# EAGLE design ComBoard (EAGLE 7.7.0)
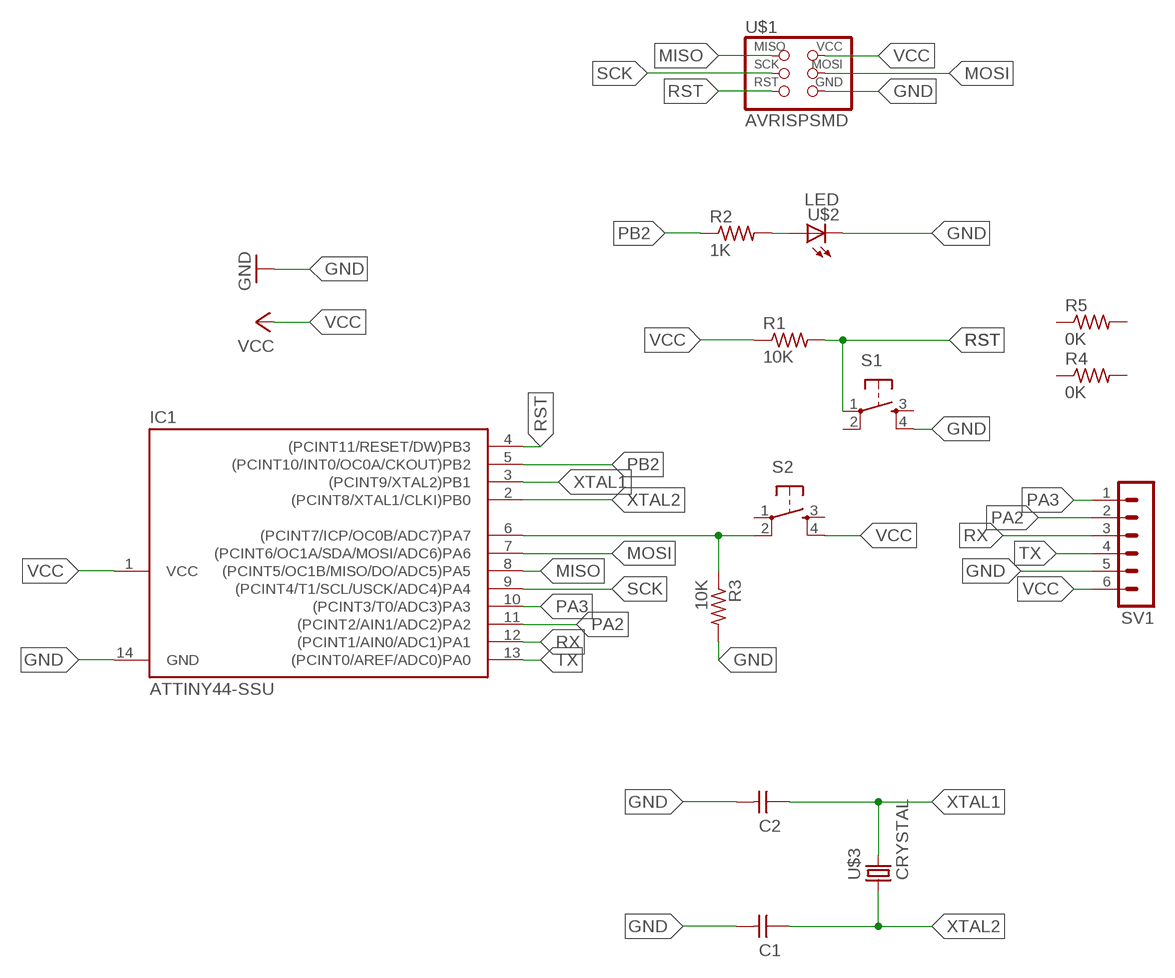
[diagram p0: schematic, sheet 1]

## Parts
C1  CAP-UNPOLARIZED  [C1206]
C2  CAP-UNPOLARIZED  [C1206]
IC1  ATTINY44-SSU  [SOIC14]
R1  10K  RES-US1206  [R1206]
R2  1K  RES-US1206  [R1206]
R3  10K  RES-US1206  [R1206]
R4  0K  RES-US1206  [R1206]
R5  0K  RES-US1206  [R1206]
S1  6MM_SWITCH6MM_SWITCH  [6MM_SWITCH]
S2  6MM_SWITCH6MM_SWITCH  [6MM_SWITCH]
SV1  MA06-1  [MA06-1]
U$1  AVRISPSMD  [2X03SMD]
U$2  LED  [LED1206]
U$3  CRYSTAL  [2-SMD-5X3MM]

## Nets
GND: C1.2 C2.2 IC1.14(GND) R3.2 S1.4(S1) SV1.5 U$1.6(GND) U$2.2(C)
MISO: IC1.8((PCINT5/OC1B/MISO/DO/ADC5)PA5) U$1.1(MISO)
MOSI: IC1.7((PCINT6/OC1A/SDA/MOSI/ADC6)PA6) U$1.4(MOSI)
N$1: R2.2 U$2.1(A)
N$2: IC1.6((PCINT7/ICP/OC0B/ADC7)PA7) R3.1 S2.2(P1)
PA2: IC1.11((PCINT2/AIN1/ADC2)PA2) SV1.2
PA3: IC1.10((PCINT3/T0/ADC3)PA3) SV1.1
PB2: IC1.5((PCINT10/INT0/OC0A/CKOUT)PB2) R2.1
RST: IC1.4((PCINT11/RESET/DW)PB3) R1.2 S1.1(P) U$1.5(RST)
RX: IC1.12((PCINT1/AIN0/ADC1)PA1) SV1.3
SCK: IC1.9((PCINT4/T1/SCL/USCK/ADC4)PA4) U$1.3(SCK)
TX: IC1.13((PCINT0/AREF/ADC0)PA0) SV1.4
VCC: IC1.1(VCC) R1.1 S2.4(S1) SV1.6 U$1.2(VCC)
XTAL1: C2.1 IC1.3((PCINT9/XTAL2)PB1) U$3.P$2
XTAL2: C1.1 IC1.2((PCINT8/XTAL1/CLKI)PB0) U$3.P$1
Unconnected: R4.1 R4.2 R5.1 R5.2 S1.2(P1) S1.3(S) S2.1(P) S2.3(S)

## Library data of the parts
C1 C2 = fab:CAP-UNPOLARIZED
IC1 = fab:ATTINY44
R1-R5 = fab:RES-US: Resistor (US Symbol)
S1 S2 = fab:6MM_SWITCH: OMRON SWITCH
SV1 = con-lstb:MA06-1: PIN HEADER; OC_FARNELL: unknown; OC_NEWARK: unknown
U$1 = fab:AVRISP
U$2 = fab:LED: LED
U$3 = fab:CRYSTAL

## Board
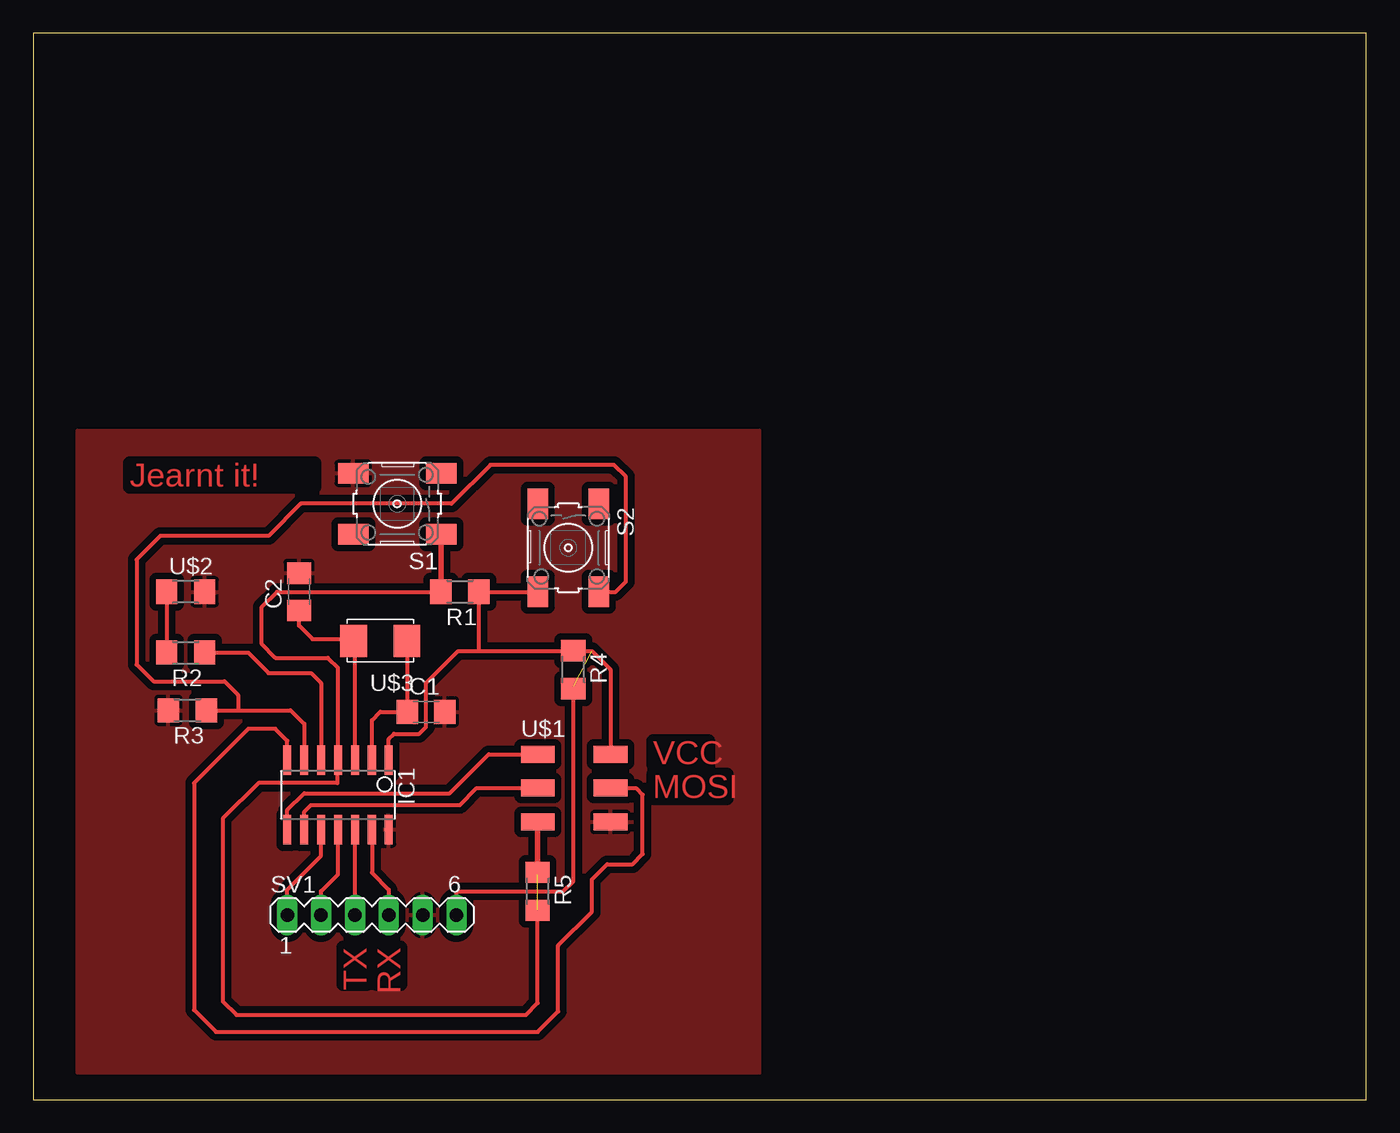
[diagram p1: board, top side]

Size 100 x 80 mm. Coordinates in mm from the lower left corner, seen from the top.
Outline: 0,0 100,0 100,80 0,80 0,0
Copper layers (1*16): Top 0.035mm / dielectric 1.5mm / Bottom 0.035mm
Design rules "default": minimum track width 10mil, minimum drill 24mil, track to track 8mil, track to pad 8mil, pad to pad 8mil, via to via 8mil, smd to smd 8mil, copper to edge 40mil, drill to drill 8mil, minimum pad ring 10mil, minimum via ring 8mil, stop-mask expansion 4mil, vias tented up to drill 0mil, thermal gap 10mil

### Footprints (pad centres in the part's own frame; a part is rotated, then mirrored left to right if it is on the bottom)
C1206 = smd 1.6 x 1.8: 1 -1.4,0; 2 1.4,0
SOIC14 = smd 0.61 x 2.21: 1 -3.81,-2.603; 2 -2.54,-2.603; 3 -1.27,-2.603; 4 0,-2.603; 5 1.27,-2.603; 6 2.54,-2.603; 7 3.81,-2.603; 8 3.81,2.603; 9 2.54,2.603; 10 1.27,2.603; 11 0,2.603; 12 -1.27,2.603; 13 -2.54,2.603; 14 -3.81,2.603
R1206 = smd 1.6 x 1.803: 1 -1.422,0; 2 1.422,0
6MM_SWITCH = smd 2.286 x 1.524: 1 -3.302,2.286; 2 3.302,2.286; 3 -3.302,-2.286; 4 3.302,-2.286
MA06-1 = drill 1.016 long: 1 -6.35,0; 2 -3.81,0; 3 -1.27,0; 4 1.27,0; 5 3.81,0; 6 6.35,0
2X03SMD = smd 2.54 x 1.27: 1 -2.54,2.54; 2 2.92,2.54; 3 -2.54,0; 4 2.92,0; 5 -2.54,-2.54; 6 2.92,-2.54
LED1206 = smd 1.6 x 1.803: 1 -1.422,0; 2 1.422,0
2-SMD-5X3MM = smd 2 x 2.4: P$1 -2,0; P$2 2,0

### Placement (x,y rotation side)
C1  29.46,29.08 0 top
C2  19.94,38.1 90 top
IC1  22.86,22.86 180 top
R1  32,38.1 180 top
R2  11.43,33.53 180 top
R3  11.56,29.21 180 top
R4  40.51,32.26 270 top
R5  37.85,15.62 270 top
S1  27.3,44.7 180 top
S2  40.13,41.4 270 top
SV1  25.4,13.84 0 top
U$1  40.39,23.37 0 top
U$2  11.43,38.1 0 top
U$3  26.04,34.42 180 top

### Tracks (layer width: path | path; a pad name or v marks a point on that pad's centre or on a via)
GND
  pour Top (isolate 0.508): 3.3,50.16 3.3,2.03 54.48,2.03 54.48,50.16
MISO
  Top 0.305: IC1.8 19.05,21.72 20.32,22.99 31.24,22.99 34.16,25.91 U$1.1
MOSI
  Top 0.305: 43.43,23.5 43.56,23.37 45.21,23.37 45.72,22.86 45.72,18.41 44.96,17.65 43.05,17.65 41.91,16.51 41.91,14.1 39.37,11.56 39.37,6.6 37.85,5.08 13.72,5.08 12.06,6.73 12.06,23.75 16.13,27.81 18.16,27.81 19.05,26.92 IC1.7
  Top 0.406: U$1.4 43.43,23.5
N$1
  Top 0.305: U$2.1 R2.2
N$2
  Top 0.305: R3.1 15.37,29.21 | 15.37,29.21 19.3,29.21 20.32,28.19 IC1.6 | S2.2 43.69,38.1 44.45,38.86 44.45,46.74 43.56,47.62 34.29,47.62 31.37,44.7 20.07,44.7 17.65,42.29 9.53,42.29 7.75,40.51 7.75,32.64 9.02,31.37 14.35,31.37 15.37,30.35 15.37,29.21
  Top 0.406: R3.1 12.95,29.18
PA2
  Top 0.305: SV1.2 21.59,15.62 22.86,16.89 IC1.11
PA3
  Top 0.305: SV1.1 19.05,15.75 21.59,18.29 IC1.10
PB2
  Top 0.305: R2.1 16.13,33.53 17.65,32 20.83,32 21.59,31.24 IC1.5
RST  (1 unrouted)
  Top 0.305: R1.2 18.29,38.1 17.14,36.96 17.14,34.16 18.16,33.15 22.1,33.15 22.86,32.38 IC1.4 22.8,25.4 22.8,23.75 16.89,23.75 14.22,21.08 14.22,7.37 15.24,6.35 36.96,6.35 37.85,7.24 37.85,14.22
  Top 0.406: R1.2 30.61,38.1 S1.1 | U$1.5 37.85,16.89
RX
  Top 0.305: SV1.3 IC1.12
SCK
  Top 0.305: IC1.9 20.32,21.59 20.83,22.1 32,22.1 33.27,23.37 U$1.3
TX
  Top 0.305: IC1.13 25.4,17.02 26.67,15.75 SV1.4
VCC  (1 unrouted)
  Top 0.305: SV1.6 31.75,15.49 31.88,15.62 39.75,15.62 40.51,16.38 40.51,30.99 | 26.73,25.53 26.67,25.59 26.67,27.05 27.05,27.43 28.96,27.43 29.46,27.94 29.46,31.24 31.88,33.66 33.4,33.66 | 33.4,33.66 41.91,33.66 43.31,32.26 U$1.2 | R1.1 S2.4 | 33.27,37.95 33.4,37.82 33.4,33.66
  Top 0.406: IC1.1 26.73,25.53 | R1.1 33.27,37.95
XTAL1
  Top 0.305: 23.91,34.54 20.95,34.54 19.94,35.56 C2.1 | IC1.3 24.13,34.32
  Top 0.406: U$3.P$2 24,34.38 | 23.91,34.54 U$3.P$2 | 24.13,34.32 U$3.P$2
XTAL2
  Top 0.305: IC1.2 25.4,28.45 26.04,29.08 C1.1 28.06,34.39
  Top 0.406: IC1.2 | U$3.P$1 28.07,34.38 | 28.19,34.26 U$3.P$1 | 28.06,34.39 U$3.P$1

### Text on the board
Top: Jearnt it! | VCC | MOSI | TX | RX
